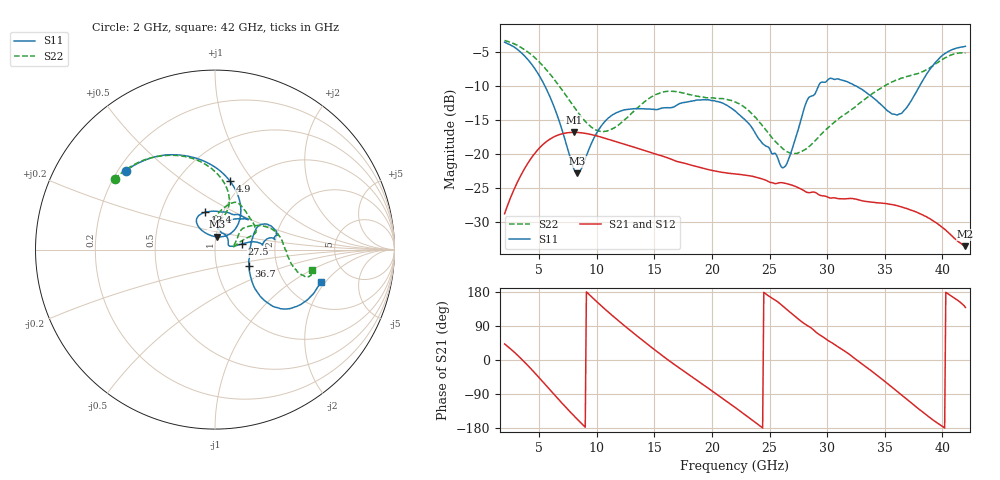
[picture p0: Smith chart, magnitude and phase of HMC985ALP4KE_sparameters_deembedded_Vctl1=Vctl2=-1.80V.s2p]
!s2p File: Measurements: S11, S21, S12, S22
# GHz S dB R 50.0
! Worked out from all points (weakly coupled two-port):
!   401 points, 2 GHz to 42 GHz, reference 50 ohm
!   highest |S21| = -16.83 dB at 8 GHz (marker M1); lowest = -33.6 dB at 42 GHz (marker M2)
!   lowest |S11| = -22.9 dB at 8.3 GHz (marker M3), VSWR 1.15, Z = 50.4 + j7.21 ohm
!   |S11| at or under -10 dB: 5.493 GHz to 29.25 GHz (23.76 GHz wide, 137 % of centre); 32.51 GHz to 38.02 GHz (5.515 GHz wide, 15.6 % of centre)
!   |S22| runs from -20.0 to -3.3 dB; largest |S21 - S12| = 0.00015
!   S11 on the Smith chart (normalised r, x): 2 GHz: 0.23, +0.36; 4.9 GHz: 0.86, +0.77; 13.4 GHz: 0.83, +0.36; 27.5 GHz: 1.35, +0.08; 36.7 GHz: 1.44, -0.27; 42 GHz: 3.12, -1.81
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2  -3.56 138.4  -28.81 42.4  -28.81 42.4  -3.30 144.9
3.4  -5.04 109.9  -23.20 4.4  -23.20 4.5  -4.31 121.5
4.9  -8.18 77.6  -19.36 -43.4  -19.36 -43.4  -6.28 97.5
6.2  -12.66 52.6  -17.57 -87.6  -17.57 -87.7  -8.80 80.7
8  -22.19 66.1  -16.83 -146.7  -16.83 -146.8  -13.02 72.7
8.3  -22.89 82.6  -16.84 -156.1  -16.85 -156.1  -13.72 73.8
8.7  -22.07 103.3  -16.91 -168.3  -16.91 -168.3  -14.62 76.3
10.7  -15.24 125.1  -17.69 134.6  -17.70 134.6  -16.69 94.0
13.4  -13.34 104.6  -19.10 65.8  -19.11 65.8  -13.43 83.0
15.4  -13.41 78.6  -20.18 18.4  -20.18 18.4  -11.08 69.5
18.9  -12.08 43.1  -21.98 -57.9  -21.99 -57.9  -11.57 43.8
22  -13.67 55.6  -22.95 -125.0  -22.96 -125.0  -12.34 22.1
24.5  -18.63 82.1  -23.77 178.4  -23.77 178.5  -16.08 18.0
26.1  -22.03 20.9  -24.25 143.6  -24.25 143.5  -19.16 9.9
27.5  -16.35 11.7  -24.99 107.9  -25.00 107.9  -19.84 8.2
28.7  -11.47 5.7  -25.63 82.3  -25.64 82.4  -18.48 18.4
31.1  -9.06 17.9  -26.60 31.7  -26.60 31.8  -14.70 37.0
33.3  -10.85 28.7  -26.99 -16.5  -27.00 -16.5  -11.95 31.8
35.4  -13.84 8.7  -27.41 -66.2  -27.41 -66.2  -9.62 20.9
36.7  -13.56 -25.0  -27.95 -98.3  -27.95 -98.3  -8.74 12.1
39.6  -6.17 -42.0  -30.30 -167.0  -30.32 -167.0  -6.56 -14.6
42  -4.17 -16.8  -33.59 138.5  -33.58 138.6  -5.17 -11.7
